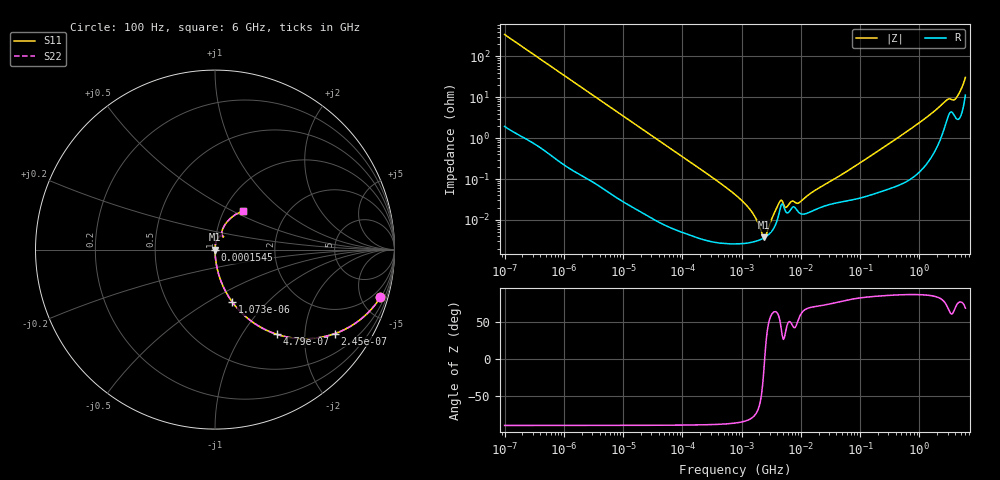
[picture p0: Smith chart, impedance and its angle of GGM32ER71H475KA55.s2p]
!Murata Part Number: GGM32ER71H475KA55
!These Parameters are Measured in Series Mode Connection
!Data Generated on Jun 19, 2026
!  o--ll--o
!Port1  Port2
!  o------o
!Operation Temp=25[degC], DC Bias Voltage=0[V]
!Freq. Start=100[Hz] Stop=6[GHz] 401[Steps]
# Hz S RI R 50
!Freq.(Hz) S11(Real) S11(Imag) S21(Real) S21(Imag) S12(Real) S12(Imag) S22(Real) S22(Imag)
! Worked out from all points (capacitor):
!   401 points, 100 Hz to 6 GHz, reference 50 ohm
!   read as one part in series: C = 4.6 uF near 109 Hz
!   lowest |Z| = 3.77 mohm at 2.373 MHz (marker M1)
!   series resonance near 2.455 MHz, so ESL is about 910 pH
!   S11 on the Smith chart (normalised r, x): 100 Hz: 1.04, -6.91; 245 Hz: 1.02, -2.83; 479 Hz: 1.01, -1.45; 1.073 kHz: 1.00, -0.65; 154.5 kHz: 1.00, -0.00; 6 GHz: 1.23, +0.57
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100  0.9214 -0.2663  0.0786 0.2663  0.0786 0.2663  0.9214 -0.2663
245  0.6659 -0.4685  0.3341 0.4685  0.3341 0.4685  0.6659 -0.4685
479  0.3457 -0.4722  0.6543 0.4722  0.6543 0.4722  0.3457 -0.4722
1073  0.097 -0.2928  0.903 0.2928  0.903 0.2928  0.097 -0.2928
2008  0.0305 -0.1685  0.9695 0.1685  0.9695 0.1685  0.0305 -0.1685
6433  0.00339 -0.0544  0.9966 0.0544  0.9966 0.0544  0.00339 -0.0544
40335  0.000165 -0.00879  0.9998 0.00879  0.9998 0.00879  0.000165 -0.00879
154540  4.47e-05 -0.0023  1 0.0023  1 0.0023  4.47e-05 -0.0023
774597  2.62e-05 -0.000419  1 0.000419  1 0.000419  2.62e-05 -0.000419
1212075  2.71e-05 -0.000227  1 0.000227  1 0.000227  2.71e-05 -0.000227
1813585  3.07e-05 -9.26e-05  1 9.26e-05  1 9.26e-05  3.07e-05 -9.26e-05
2372521  3.62e-05 -1.06e-05  1 1.06e-05  1 1.06e-05  3.62e-05 -1.06e-05
3103719  4.95e-05 7.75e-05  1 -7.75e-05  1 -7.75e-05  4.95e-05 7.75e-05
4440638  0.000179 0.000223  0.9998 -0.000223  0.9998 -0.000223  0.000179 0.000223
5809218  0.000149 0.000145  0.9999 -0.000145  0.9999 -0.000145  0.000149 0.000145
6948629  0.000192 0.00021  0.9998 -0.00021  0.9998 -0.00021  0.000192 0.00021
9090158  0.000157 0.000206  0.9998 -0.000206  0.9998 -0.000206  0.000157 0.000206
1.555665e7  0.000165 0.000448  0.9998 -0.000448  0.9998 -0.000448  0.000165 0.000448
3.124326e8  0.000633 0.00741  0.9994 -0.00741  0.9994 -0.00741  0.000633 0.00741
2.802721e9  0.028 0.0752  0.972 -0.0752  0.972 -0.0752  0.028 0.0752
4.009986e9  0.0384 0.0773  0.9616 -0.0773  0.9616 -0.0773  0.0384 0.0773
6e9  0.1579 0.2164  0.8421 -0.2164  0.8421 -0.2164  0.1579 0.2164
